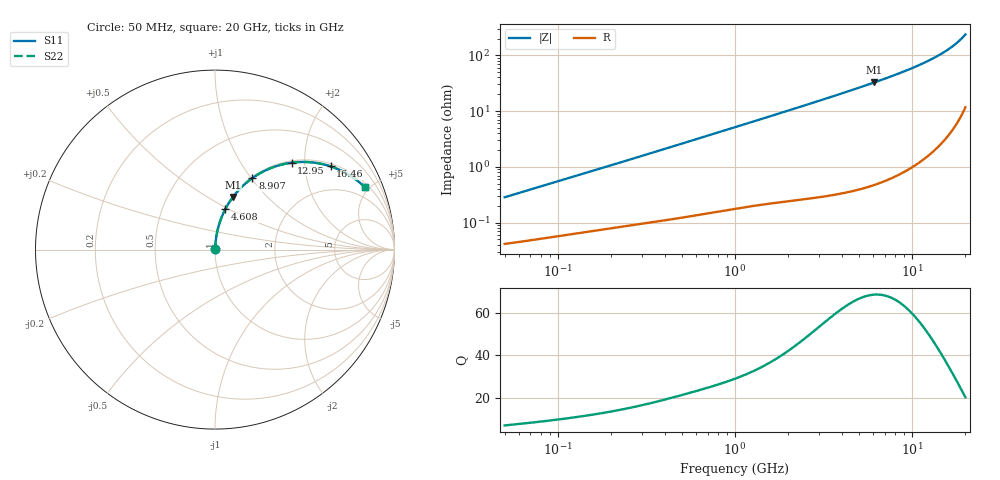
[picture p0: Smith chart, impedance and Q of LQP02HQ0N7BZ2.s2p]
!Murata Part Number: LQP02HQ0N7BZ2
!These Parameters are Measured in Series Mode Connection
!  o--[Z]--o
!Port1  Port2
!  o-------o
!Freq. Start=50[MHz] Stop=20[GHz], 401[Steps]
# Hz S RI R 50
!Freq.(Hz) S11(Real) S11(Imag) S21(Real) S21(Imag) S12(Real) S12(Imag) S22(Real) S22(Imag)
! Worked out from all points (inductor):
!   401 points, 50 MHz to 20 GHz, reference 50 ohm
!   read as one part in series: L = 888 pH near 51.52 MHz
!   highest Q = 68.9 at 6.125 GHz (marker M1), where L = 848 pH
!   S11 on the Smith chart (normalised r, x): 50 MHz: 1.00, +0.01; 4.608 GHz: 1.01, +0.48; 8.907 GHz: 1.02, +1.01; 12.95 GHz: 1.04, +1.72; 16.46 GHz: 1.08, +2.71; 20 GHz: 1.23, +4.72
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5e7  0.000423 0.00282  0.9996 -0.00282  0.9996 -0.00282  0.000423 0.00282
5.152053e7  0.000429 0.0029  0.9996 -0.0029  0.9996 -0.0029  0.000429 0.0029
1.364002e8  0.000717 0.00737  0.9993 -0.00737  0.9993 -0.00737  0.000717 0.00737
3.721004e8  0.00144 0.0194  0.9986 -0.0194  0.9986 -0.0194  0.00144 0.0194
6.380365e8  0.00248 0.0329  0.9975 -0.0329  0.9975 -0.0329  0.00248 0.0329
1e9  0.00438 0.051  0.9956 -0.051  0.9956 -0.051  0.00438 0.051
1.714689e9  0.00982 0.0865  0.9902 -0.0865  0.9902 -0.0865  0.00982 0.0865
2.728004e9  0.0217 0.1361  0.9783 -0.1361  0.9783 -0.1361  0.0217 0.1361
3.572216e9  0.0355 0.1767  0.9645 -0.1767  0.9645 -0.1767  0.0355 0.1767
4.608136e9  0.0575 0.2253  0.9425 -0.2253  0.9425 -0.2253  0.0575 0.2253
6.125241e9  0.0998 0.2925  0.9002 -0.2925  0.9002 -0.2925  0.0998 0.2925
7.442007e9  0.1461 0.346  0.8539 -0.346  0.8539 -0.346  0.1461 0.346
8.907419e9  0.208 0.3981  0.792 -0.3981  0.792 -0.3981  0.208 0.3981
9.892087e9  0.2553 0.4278  0.7447 -0.4278  0.7447 -0.4278  0.2553 0.4278
1.082228e10  0.3038 0.4512  0.6962 -0.4512  0.6962 -0.4512  0.3038 0.4512
1.183995e10  0.3607 0.4708  0.6393 -0.4708  0.6393 -0.4708  0.3607 0.4708
1.295331e10  0.4265 0.4842  0.5735 -0.4842  0.5735 -0.4842  0.4265 0.4842
1.482269e10  0.5422 0.4858  0.4578 -0.4858  0.4578 -0.4858  0.5422 0.4858
1.646126e10  0.6438 0.4641  0.3562 -0.4641  0.3562 -0.4641  0.6438 0.4641
1.800918e10  0.7346 0.4236  0.2654 -0.4236  0.2654 -0.4236  0.7346 0.4236
1.940974e10  0.8083 0.3718  0.1917 -0.3718  0.1917 -0.3718  0.8083 0.3718
2e10  0.8361 0.3462  0.1639 -0.3462  0.1639 -0.3462  0.8361 0.3462
